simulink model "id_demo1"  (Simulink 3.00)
settings: Solver=ode45  SolverMode=SingleTasking  StartTime=0.0  StopTime=10  RelTol=1e-3  AbsTol=1e-3
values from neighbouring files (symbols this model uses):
  Au = [a0 a1;a2]    [data_id1.m]    (also in data_id2.m = [a0;[a1 a2]])
  Ay = [A0 A1;A2]    [data_id1.m]    (also in data_id2.m = A0)
  Bu = [b0;b1]    [data_id1.m]    (also in data_id2.m)
  By = [B0;B1]    [data_id1.m]    (also in data_id2.m)
  Cu = [c0 c1]/den(1)    [data_id1.m]    (also in data_id2.m = [c0 c1])
  Cy = [C0;C1]/den(1)    [data_id1.m]    (also in data_id2.m = [C0;C1])
  Du = zeros(in*(cit+1),in)    [data_id1.m]    (also in data_id2.m = zeros(cit*in,in))
  Dy = -[zeros(out,out);By]/den(1)    [data_id1.m]    (also in data_id2.m = [D1;D2])
libraries: simulink3 x1

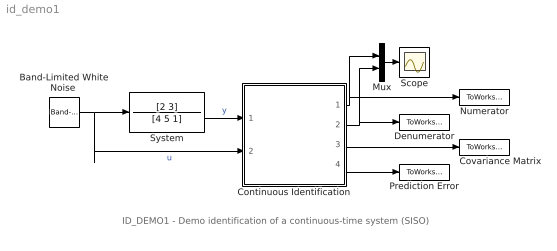
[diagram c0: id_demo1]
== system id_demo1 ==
  note: ID_DEMO1 - Demo identification of a continuous-time system (SISO)
  "Band-Limited White Noise " : simulink3/Sources/Band-Limited White Noise  Cov=[0.1]  Ts=0.1  seed=[23341]
  Continuous Identification : Subsystem  mask(Continuous Identification){par1=[1,2], tc=[0.5], par2=[0.985,0.01], poc=[0 0 0 0], kov=[10e6], ts=[1]}
      mask prompts: par1 "Degrees of numerator and denominator -  [dn, dd]:"; tc "Time constant of the filter - [Tc]:"; par2 "Exponential forgetting and Bittanti's correction - [L, d]:"; poc "Initial parameter estimates - [theta(1) ... theta(n)]:"; kov "Covariance matrix (see help, standard - [10e6]):"; ts "Sampling time - [ts]:"
      mask help: Continuous identification Authors: Lubos Cirka and Miroslav Fikar 1998 - 2004
      mask init:
      | cit=par1(1);men=par1(2);L=par2(1);d=par2(2); n=cit+men+1;m=1;in=1;out=1;eval('data_id1');
  Covariance Matrix : ToWorkspace  VariableName=CovMatrix  SampleTime=0  SaveFormat=Matrix
  Denumerator : ToWorkspace  VariableName=A  SampleTime=0  SaveFormat=Matrix
  Mux : Mux  Inputs=2
  Numerator : ToWorkspace  VariableName=B  SampleTime=0  SaveFormat=Matrix
  Prediction Error : ToWorkspace  VariableName=PredError  SampleTime=0  SaveFormat=Matrix
  Scope : Scope
  System : TransferFcn  Numerator=[2 3]  Denominator=[4 5 1]
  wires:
  System/1 -> Continuous Identification/1(y)  "y"
  "Band-Limited White Noise "/1 -> System/1, Continuous Identification/2(u)  "u"
  Continuous Identification/3("Covariance matrix ") -> Covariance Matrix/1
  Continuous Identification/4(prediction error) -> Prediction Error/1
  Mux/1 -> Scope/1
  Continuous Identification/1(B) -> Numerator/1, Mux/1
  Continuous Identification/2(A) -> Denumerator/1, Mux/2

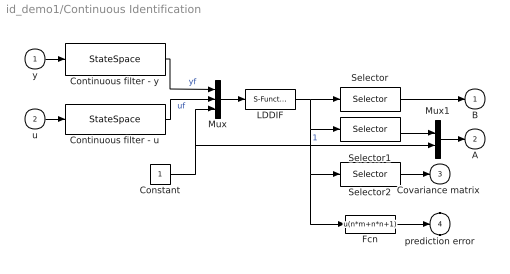
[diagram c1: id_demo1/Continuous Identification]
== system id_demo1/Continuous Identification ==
  y : Inport  Port=1  PortWidth=-1  SampleTime=-1  DataType=auto
  u : Inport  Port=2  PortWidth=-1  SampleTime=-1  DataType=auto
  Constant : Constant  Value=1
  Continuous filter - u : StateSpace  A=Au  B=Bu  C=Cu  D=Du  X0=0
  Continuous filter - y : StateSpace  A=Ay  B=By  C=Cy  D=Dy  X0=0
  Fcn : Fcn  Expr=u(n*m+n*n+1)
  LDDIF : S-Function  FunctionName=lddif_s  Parameters=m ,n+1 ,L ,d, [poc 0], kov, ts  PortCounts=[]  SFunctionModules=''
  Mux : Mux  Inputs=3
  Mux1 : Mux  Inputs=2
  Selector : Selector  Elements=[men+cit+1:-1:men+1]  InputPortWidth=(n+1)*m+(n+1)*(n+1)+m
  Selector1 : Selector  Elements=[men:-1:1]  InputPortWidth=(n+1)*m+(n+1)*(n+1)+m
  Selector2 : Selector  Elements=[(n+1)*m+1:1:(n+1)*m+(n+1)*(n+1)]  InputPortWidth=(n+1)*m+(n+1)*(n+1)+m
  B : Outport  Port=1  InitialOutput=0
  A : Outport  Port=2  InitialOutput=0
  "Covariance matrix " : Outport  Port=3  InitialOutput=0
  prediction error : Outport  Port=4  InitialOutput=0
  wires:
  LDDIF/1 -> Selector/1, Selector1/1, Selector2/1, Fcn/1
  Continuous filter - u/1 -> Mux/2  "uf"
  Continuous filter - y/1 -> Mux/1  "yf"
  u/1 -> Continuous filter - u/1
  y/1 -> Continuous filter - y/1
  Selector/1 -> B/1
  Mux/1 -> LDDIF/1
  Constant/1 -> Mux/3, Mux1/2  "1"
  Selector1/1 -> Mux1/1
  Mux1/1 -> A/1
  Selector2/1 -> "Covariance matrix "/1
  Fcn/1 -> prediction error/1
